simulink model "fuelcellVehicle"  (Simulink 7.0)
settings: Solver=ode45  StartTime=0.0  StopTime=10.0  RelTol=1e-3
InitFcn:
  | t_Start=tic;
StopFcn:
  | t_elapsed=toc(t_Start);
  | fuel_cons=(1000*(fueltank_simple1_std(end,1)/fueltank_simple1_std(end,3)))/(chassis_simple4_std(end,2)/100000);
  | 
  | disp(' ')
  | disp(['Time Elapsed: ' num2str(round(100*t_elapsed)/100) 's'])
  | disp(['Fuel Consumption: ' num2str(round(1000*fuel_cons)/1000) 'L/100km'])
undefined symbols (not defined in the file or in its folder): computed_mass, DC, fuelcellVehicle, Left, levelinit, slcm
libraries: simulink x11
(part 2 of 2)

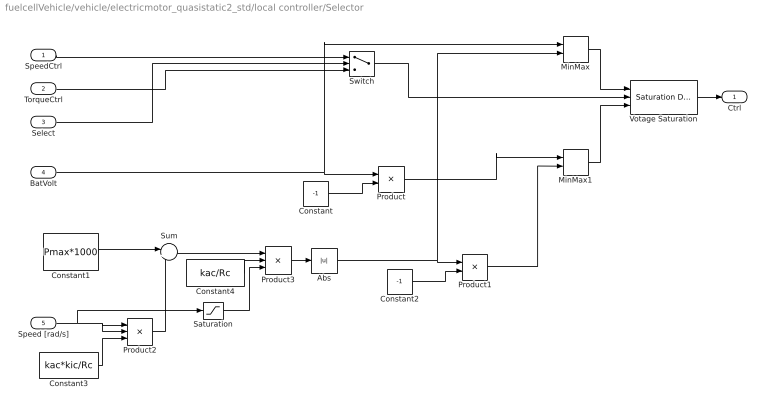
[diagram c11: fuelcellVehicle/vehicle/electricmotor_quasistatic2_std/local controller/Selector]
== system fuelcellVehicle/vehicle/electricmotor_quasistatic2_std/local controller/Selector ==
  SpeedCtrl : Inport  OutDataType=sfix(16)  OutScaling=2^0
  TorqueCtrl : Inport  Port=2  OutDataType=sfix(16)  OutScaling=2^0
  Select : Inport  Port=3  OutDataType=sfix(16)  OutScaling=2^0
  BatVolt : Inport  Port=4  OutDataType=sfix(16)  OutScaling=2^0
  Speed [rad/s] : Inport  Port=5  OutDataType=sfix(16)  OutScaling=2^0
  Abs : Abs
  Constant : Constant  Value=-1  OutDataType=sfix(16)  OutScaling=2^0
  Constant1 : Constant  Value=Pmax*1000  OutDataType=sfix(16)  OutScaling=2^0
  Constant2 : Constant  Value=-1  OutDataType=sfix(16)  OutScaling=2^0
  Constant3 : Constant  Value=kac*kic/Rc  OutDataType=sfix(16)  OutScaling=2^0
  Constant4 : Constant  Value=kac/Rc  OutDataType=sfix(16)  OutScaling=2^0
  MinMax : MinMax  Inputs=2  OutDataType=sfix(16)  OutScaling=2^0
  MinMax1 : MinMax  Function=max  Inputs=2  OutDataType=sfix(16)  OutScaling=2^0
  Product : Product  OutDataType=sfix(16)  OutScaling=2^0
  Product1 : Product  OutDataType=sfix(16)  OutScaling=2^0
  Product2 : Product  Inputs=***  OutDataType=sfix(16)  OutScaling=2^0
  Product3 : Product  Inputs=*/*  OutDataType=sfix(16)  OutScaling=2^0
  Saturation : Saturate  UpperLimit=inf  LowerLimit=0.1
  Sum : Sum  Inputs=|++  OutDataType=sfix(16)  OutScaling=2^0
  Switch : Switch  Threshold=0.5
  Votage Saturation : simulink/Discontinuities/Saturation Dynamic  SystemSampleTime=-1  OutMin=[]  OutMax=[]  OutDataTypeStr=Inherit: Same as second input  OutDataType=sfix(16)  OutScaling=2^-10  DoSatur=off
  Ctrl : Outport  OutDataType=sfix(16)  OutScaling=2^0
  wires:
  Select/1 -> Switch/2
  TorqueCtrl/1 -> Switch/3
  SpeedCtrl/1 -> Switch/1
  Switch/1 -> Votage Saturation/2
  BatVolt/1 -> Product/1, MinMax/1
  Constant/1 -> Product/2
  Votage Saturation/1 -> Ctrl/1
  MinMax/1 -> Votage Saturation/1
  Constant2/1 -> Product1/2
  Abs/1 -> MinMax/2, Product1/1
  MinMax1/1 -> Votage Saturation/3
  Product/1 -> MinMax1/1
  Product1/1 -> MinMax1/2
  Speed [rad/s]/1 -> Product2/1, Product2/2, Saturation/1
  Constant1/1 -> Sum/1
  Constant3/1 -> Product2/3
  Sum/1 -> Product3/1
  Constant4/1 -> Product3/2
  Product3/1 -> Abs/1
  Product2/1 -> Sum/2
  Saturation/1 -> Product3/3

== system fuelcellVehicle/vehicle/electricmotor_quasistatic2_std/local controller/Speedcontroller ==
  Speedref : Inport  OutDataType=sfix(16)  OutScaling=2^0
  Speed : Inport  Port=2  OutDataType=sfix(16)  OutScaling=2^0
  Gain : Gain  Gain=Kp  ParameterDataType=sfix(16)  ParameterScaling=2^0  OutDataType=sfix(16)  OutScaling=2^0
  Gain1 : Gain  Gain=Ki  ParameterDataType=sfix(16)  ParameterScaling=2^0  OutDataType=sfix(16)  OutScaling=2^0
  Gain2 : Gain  Gain=Rc/kac  ParameterDataType=sfix(16)  ParameterScaling=2^0  OutDataType=sfix(16)  OutScaling=2^0
  Gain3 : Gain  Gain=kic  ParameterDataType=sfix(16)  ParameterScaling=2^0  OutDataType=sfix(16)  OutScaling=2^0
  "Generator? : -1 " : Gain  ParameterDataType=sfix(16)  ParameterScaling=2^0  OutDataType=sfix(16)  OutScaling=2^0
  "Generator? : -1  " : Gain  Orientation=up  ParameterDataType=sfix(16)  ParameterScaling=2^0  OutDataType=sfix(16)  OutScaling=2^0
  Integrator : Integrator
  Sum : Sum  Inputs=|++  OutDataType=sfix(16)  OutScaling=2^0
  Sum1 : Sum  Inputs=|+-  OutDataType=sfix(16)  OutScaling=2^0
  Sum2 : Sum  Inputs=|++  OutDataType=sfix(16)  OutScaling=2^0
  Volt : Outport  OutDataType=sfix(16)  OutScaling=2^0
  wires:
  Gain/1 -> Sum/1
  Integrator/1 -> Sum/2
  Gain1/1 -> Integrator/1
  Speedref/1 -> Sum1/1
  Speed/1 -> Gain3/1, Sum1/2
  Sum1/1 -> Gain/1, Gain1/1
  Sum2/1 -> Volt/1  "compensated voltage"
  Gain2/1 -> Sum2/1
  Gain3/1 -> "Generator? : -1  "/1
  Sum/1 -> "Generator? : -1 "/1  "desired torque"
  "Generator? : -1 "/1 -> Gain2/1
  "Generator? : -1  "/1 -> Sum2/2

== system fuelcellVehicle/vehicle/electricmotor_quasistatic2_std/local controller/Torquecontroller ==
  Torqueref : Inport  OutDataType=sfix(16)  OutScaling=2^0
  Speed : Inport  Port=2  OutDataType=sfix(16)  OutScaling=2^0
  Gain : Gain  Gain=Rc/kac  ParameterDataType=sfix(16)  ParameterScaling=2^0  OutDataType=sfix(16)  OutScaling=2^0
  Gain1 : Gain  Gain=kic  ParameterDataType=sfix(16)  ParameterScaling=2^0  OutDataType=sfix(16)  OutScaling=2^0
  Sum : Sum  Inputs=|++  OutDataType=sfix(16)  OutScaling=2^0
  Volt : Outport  OutDataType=sfix(16)  OutScaling=2^0
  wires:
  Sum/1 -> Volt/1
  Gain/1 -> Sum/1
  Gain1/1 -> Sum/2
  Torqueref/1 -> Gain/1
  Speed/1 -> Gain1/1

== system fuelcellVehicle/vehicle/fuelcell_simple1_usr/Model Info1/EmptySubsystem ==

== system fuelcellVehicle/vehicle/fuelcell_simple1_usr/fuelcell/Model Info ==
  EmptySubsystem : Subsystem

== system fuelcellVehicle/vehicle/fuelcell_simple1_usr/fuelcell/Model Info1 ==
  EmptySubsystem : Subsystem

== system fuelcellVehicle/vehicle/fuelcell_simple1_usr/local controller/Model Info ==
  EmptySubsystem : Subsystem

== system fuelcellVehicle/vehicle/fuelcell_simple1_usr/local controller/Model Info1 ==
  EmptySubsystem : Subsystem

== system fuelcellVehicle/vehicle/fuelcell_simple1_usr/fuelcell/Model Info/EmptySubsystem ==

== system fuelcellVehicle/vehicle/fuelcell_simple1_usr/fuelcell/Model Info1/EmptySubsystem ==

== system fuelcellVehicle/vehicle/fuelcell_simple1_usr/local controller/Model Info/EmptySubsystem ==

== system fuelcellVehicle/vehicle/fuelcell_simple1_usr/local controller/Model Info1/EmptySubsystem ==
